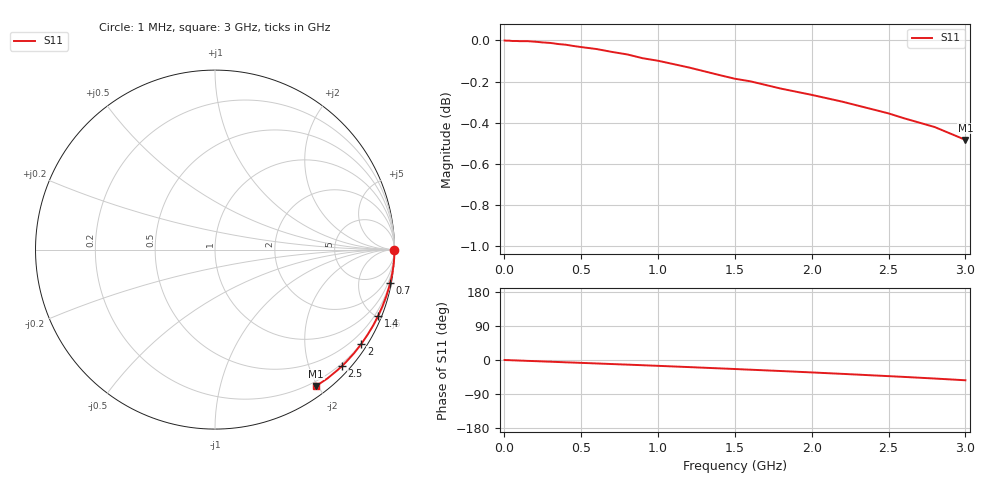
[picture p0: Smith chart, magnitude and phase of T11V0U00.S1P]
! SIEMENS Small Signal Semiconductors
! BAT68-04
! Si Schottky Diode (2 diodes in series, pin 3 open) in SOT23
! VR = 1 V
! S-Parameters:  August  1994
# GHz  S  MA  R  50
!  f  S11
! GHz  MAG  ANG
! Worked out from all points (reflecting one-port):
!   33 points, 1 MHz to 3 GHz, reference 50 ohm
!   lowest |S11| = -0.5 dB at 3 GHz (marker M1), VSWR 35.97, Z = 6.84 - j98.8 ohm
!   phase of S11 starts at 0 deg and turns -54 deg over the sweep
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0.001  1 0.0
0.003  1 0.0
0.01  0.9999 -0.2
0.03  0.9999 -0.4
0.05  0.9997 -0.8
0.06  0.9997 -0.9
0.15  0.9996 -2.3
0.2  0.9993 -3.0
0.25  0.9989 -3.8
0.3  0.9986 -4.5
0.4  0.9976 -6.1
0.45  0.9969 -6.8
0.6  0.9952 -9.1
0.7  0.9936 -10.7
0.8  0.9922 -12.2
1  0.9887 -15.4
1.2  0.985 -18.7
1.4  0.9808 -22.1
1.5  0.9788 -23.8
1.6  0.9774 -25.6
1.8  0.9734 -29.1
2  0.97 -32.8
2.2  0.9663 -36.6
2.4  0.9621 -40.6
2.5  0.96 -42.6
2.6  0.9574 -44.6
2.8  0.9527 -48.9
3  0.9459 -53.5
